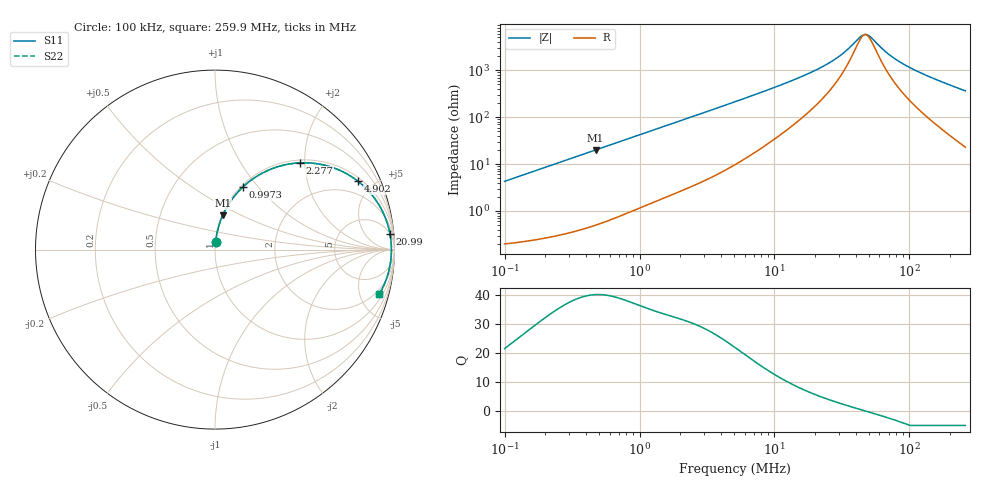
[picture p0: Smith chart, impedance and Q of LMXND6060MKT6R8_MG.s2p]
! LMXND6060MKT6R8_MG  S-PARAMETER MODEL  ( General Type )
! Model Generated by TAIYO YUDEN Corporation (http://www.ty-top.com)
! Version 1.0
! TAIYO YUDEN Control No. 191025NI43SB-FBB
! Copyright(c) 2019 TAIYO YUDEN CO.,LTD. All Rights Reserved.
! Product Description (link to TY-COMPAS)
! https://ds.yuden.co.jp/TYCOMPAS/or/detail?pn=LMXND6060MKT6R8MMG&u=M
! Products Name : Inductors
! Characteristics :
!  Inductance : 6.8 uH , SRF(min) : 30 MHz , DC Resistance(max) : 0.198 Ohm
!  Rated Current : Saturation :1300 mA , Temp Rise : 1350 mA
!  Case Size : 6.0 x 6.0 / 0.236 x 0.236 [mm/inch] , Thickness : 1.2 / 0.047 [mm/inch]
!  (Conditions: Temperature = 25 degC , DC Bias Current/Voltage = 0A / 0V)
! External Node Assignments :
!  1  o---GGG---o  2
! GND o---------o GND
! Frequency Range : 0.1MHz  -  259.929867MHz  [ 402 STEP ]
# MHz S RI R 50
! Freq[MHz].  S11 Real  S11 Imag  S21 Real  S21 Imag  S12 Real  S12 Imag  S22 Real  S22 Imag
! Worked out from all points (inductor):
!   401 points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, 100 kHz to 259.9 MHz, reference 50 ohm
!   read as one part in series: L = 6.81 uH near 104 kHz
!   highest Q = 40.2 at 472.5 kHz (marker M1), where L = 6.75 uH
!   self-resonance near 47.11 MHz
!   S11 on the Smith chart (normalised r, x): 100 kHz: 1.00, +0.09; 997.3 kHz: 1.02, +0.84; 2.277 MHz: 1.06, +1.90; 4.902 MHz: 1.18, +4.09; 20.99 MHz: 5, +21; 259.9 MHz: 1.46, -7.25
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0.1  0.00381 0.0426  0.9962 -0.0426  0.9962 -0.0426  0.00381 0.0426
0.202926  0.01 0.0855  0.99 -0.0855  0.99 -0.0855  0.01 0.0855
0.37324  0.0282 0.1534  0.9718 -0.1534  0.9718 -0.1534  0.0282 0.1534
0.472535  0.043 0.1908  0.957 -0.1908  0.957 -0.1908  0.043 0.1908
0.997345  0.1564 0.3498  0.8436 -0.3498  0.8436 -0.3498  0.1564 0.3498
1.393082  0.26 0.4242  0.74 -0.4242  0.74 -0.4242  0.26 0.4242
2.277222  0.4743 0.4834  0.5257 -0.4834  0.5257 -0.4834  0.4743 0.4834
3.243948  0.6405 0.4622  0.3595 -0.4622  0.3595 -0.4622  0.6405 0.4622
4.90178  0.7967 0.3809  0.2033 -0.3809  0.2033 -0.3809  0.7967 0.3809
5.098332  0.8084 0.3714  0.1916 -0.3714  0.1916 -0.3714  0.8084 0.3714
9.015819  0.9221 0.2345  0.0779 -0.2345  0.0779 -0.2345  0.9221 0.2345
19.02902  0.9721 0.1019  0.0279 -0.1019  0.0279 -0.1019  0.9721 0.1019
20.99434  0.9747 0.0887  0.0253 -0.0887  0.0253 -0.0887  0.9747 0.0887
30.50056  0.9809 0.0445  0.0191 -0.0445  0.0191 -0.0445  0.9809 0.0445
34.99999  0.9821 0.03  0.0179 -0.03  0.0179 -0.03  0.9821 0.03
42.60291  0.9829 0.01  0.0171 -0.01  0.0171 -0.01  0.9829 0.01
46.088  0.983 0.00218  0.017 -0.00218  0.017 -0.00218  0.983 0.00218
50.84796  0.983 -0.00761  0.017 0.00761  0.017 0.00761  0.983 -0.00761
71.02397  0.9812 -0.0419  0.0188 0.0419  0.0188 0.0419  0.9812 -0.0419
88.1685  0.9785 -0.0662  0.0215 0.0662  0.0215 0.0662  0.9785 -0.0662
118.4051  0.9719 -0.1041  0.0281 0.1041  0.0281 0.1041  0.9719 -0.1041
259.9299  0.9161 -0.2475  0.0839 0.2475  0.0839 0.2475  0.9161 -0.2475
